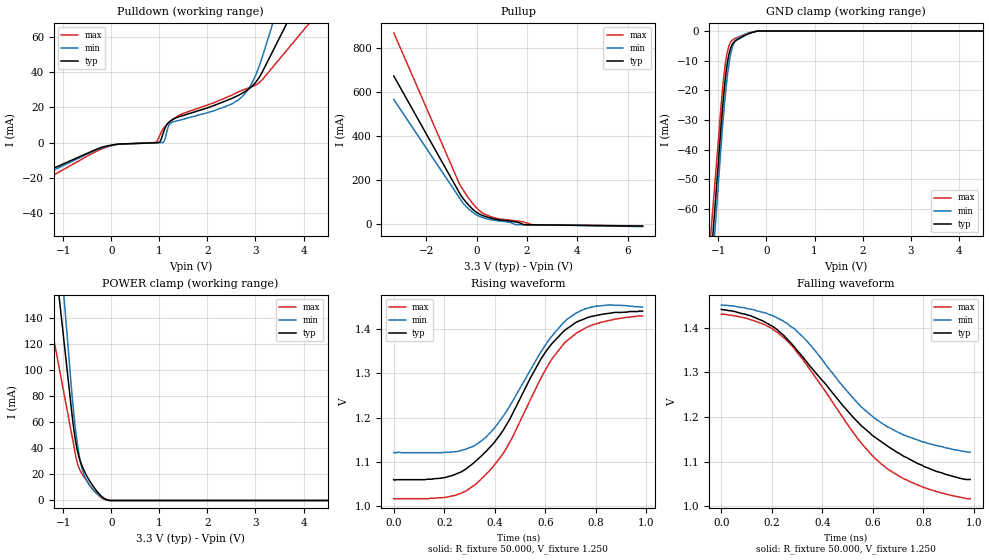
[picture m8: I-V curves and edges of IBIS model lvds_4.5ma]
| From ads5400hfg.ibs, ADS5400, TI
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[Model]   lvds_4.5ma
Model_type 3-state
Vref=1.250E+00
Rref=5.000E+01
Cref=0.000E+00
Vmeas=1.250E+00
C_comp   4.960E-13   4.830E-13   5.040E-13
[Voltage Range]   3.300E+00   3.000E+00   3.600E+00
[POWER Clamp Reference]   3.300E+00   3.000E+00   3.600E+00
[GND Clamp Reference]   0.000E+00   0.000E+00   0.000E+00
[Pullup Reference]   3.300E+00   3.000E+00   3.600E+00
[Pulldown Reference]   0.000E+00   0.000E+00   0.000E+00
[Temperature Range]   25   100   -40
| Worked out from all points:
|   slope of the pulldown table from 0 to 0.495 V, typ, clamps not added: 529 ohm
|   slope of the pullup table from 0 to 0.495 V, typ, clamps not added: 21 ohm
|   GND clamp passes 1 mA (typ) near -0.38 V on its own axis
|   POWER clamp passes 1 mA (typ) near -0.12 V on its own axis
|   rising waveform, R_fixture 50.000, V_fixture 1.250: 20-80 % time 237ps typ, 213ps min, 239ps max; typ from 1.06 V to 1.44 V
|   falling waveform, R_fixture 50.000, V_fixture 1.250: 20-80 % time 377ps typ, 319ps min, 327ps max; typ from 1.44 V to 1.06 V
[GND Clamp]
-3.3V     -537.3mA   -567.9mA   -498.8mA
-1.02V    -47.94mA   -55.46mA   -40.24mA
-940mV    -30.65mA   -37.38mA   -24.01mA
-900mV    -22.97mA   -29.21mA   -17.03mA
-860mV    -16.46mA   -22.06mA   -11.43mA
-820mV    -11.32mA   -15.91mA   -7.404mA
-780mV    -7.688mA   -10.94mA   -4.923mA
-720mV    -4.719mA   -5.907mA   -3.208mA
-620mV    -3.03mA    -2.674mA   -2.233mA
-400mV    -1.112mA   -828.3uA   -826.9uA
-160mV    0A         0A         0A
6.6V      0A         0A         0A
[Power Clamp]
-3.3V     900.2mA    1.194A     533.9mA
-900mV    92.34mA    116.4mA    64.81mA
-820mV    65.46mA    80.49mA    49.17mA
-760mV    48.47mA    58.11mA    37.01mA
-700mV    36.63mA    41.13mA    27.48mA
-640mV    29.05mA    28.44mA    22.11mA
-580mV    23.7mA     20.49mA    18.63mA
-460mV    15.3mA     11.78mA    12.25mA
-320mV    7.805mA    5.657mA    5.799mA
-160mV    1.836mA    1.349mA    1.036mA
-40mV     0A         0A         0A
6.6V      0A         0A         0A
[Pullup]
-3.3V     674.2mA    567mA      871.4mA
-700mV    143mA      120.3mA    185.1mA
-540mV    114.7mA    93.38mA    154.5mA
-320mV    84.54mA    67.21mA    116.5mA
-80mV     58.12mA    45.53mA    81.45mA
140mV     42.09mA    32.1mA     56.35mA
720mV     21.06mA    14.87mA    26.87mA
1.34V     11.8mA     5.528mA    16.09mA
1.56V     7.886mA    -4.329mA   13.1mA
1.88V     -4.459mA   -4.952mA   6.909mA
2.22V     -5.177mA   -5.316mA   -4.833mA
6.6V      -11.08mA   -13.23mA   -10.17mA
[Pulldown]
-3.3V     -39.87mA   -42.87mA   -50.56mA
-220mV    -2.851mA   -3.247mA   -3.834mA
920mV     -113.7uA   -150.5uA   25.48uA
1.02V     888.4uA    -60.63uA   4.88mA
1.08V     5.506mA    120.9uA    7.861mA
1.18V     11.06mA    8.762mA    10.9mA
1.24V     12.47mA    11.21mA    12.31mA
2.16V     21.29mA    18.3mA     22.89mA
2.7V      27.64mA    25.49mA    29.43mA
2.92V     31.76mA    33.47mA    31.61mA
3.16V     41.02mA    50.12mA    36.3mA
6.6V      227.3mA    351.6mA    148.8mA
[Rising Waveform]
R_fixture = 50.000
V_fixture = 1.250
V_fixture_min = 1.250
V_fixture_max = 1.250
|  time   V(typ)   V(min)   V(max)
0s        1.06V      1.121V     1.017V
205ps     1.065V     1.122V     1.02V
322.5ps   1.101V     1.138V     1.049V
365ps     1.124V     1.156V     1.072V
437.5ps   1.176V     1.207V     1.123V
582.5ps   1.333V     1.349V     1.289V
625ps     1.367V     1.384V     1.332V
677.5ps   1.398V     1.418V     1.37V
800ps     1.431V     1.452V     1.412V
985ps     1.441V     1.45V      1.43V
[Falling Waveform]
R_fixture = 50.000
V_fixture = 1.250
V_fixture_min = 1.250
V_fixture_max = 1.250
|  time   V(typ)   V(min)   V(max)
0s        1.441V     1.45V      1.43V
90ps      1.431V     1.445V     1.422V
167.5ps   1.414V     1.434V     1.408V
255ps     1.378V     1.411V     1.374V
337.5ps   1.324V     1.371V     1.317V
522.5ps   1.199V     1.242V     1.165V
595ps     1.16V      1.203V     1.115V
655ps     1.136V     1.179V     1.085V
802.5ps   1.089V     1.144V     1.042V
985ps     1.06V      1.121V     1.017V
[Ramp]
dV/dt_f   2.2800E-01/4.3031E-10   1.9700E-01/3.5797E-10   2.4780E-01/3.5992E-10
dV/dt_r   2.2800E-01/2.3820E-10   1.9700E-01/2.0810E-10   2.4780E-01/2.4300E-10
R_load = 50
